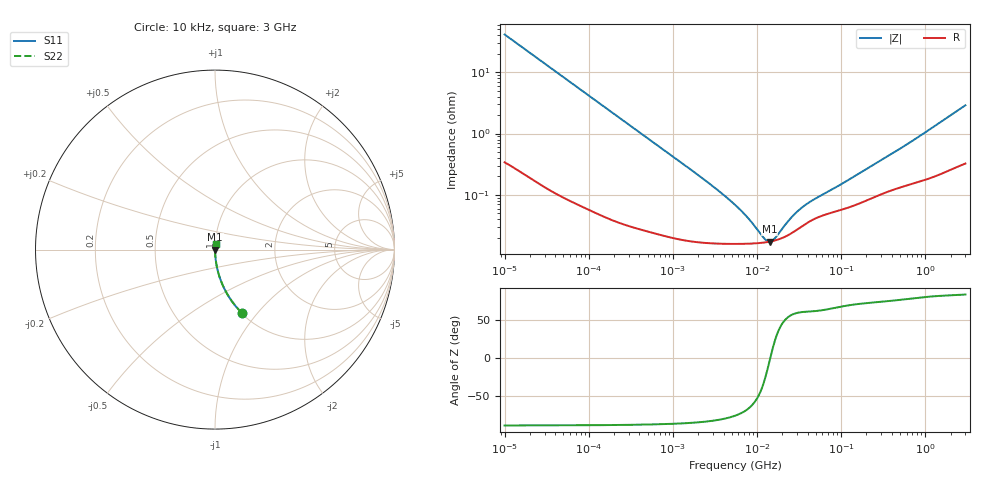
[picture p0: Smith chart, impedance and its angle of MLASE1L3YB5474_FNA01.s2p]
! MLASE1L3YB5474_FNA01  S-PARAMETER MODEL  ( Standard Model )
! Model Generated by TAIYO YUDEN Corporation (http://www.ty-top.com)
! Version 1.0
! TAIYO YUDEN Control No. 220601
! Copyright(c) 2010 TAIYO YUDEN CO.,LTD. All Rights Reserved.
! Product Description (link to TY-COMPAS)
! https://ds.yuden.co.jp/TYCOMPAS/or/detail?pn=MLASE1L3YB5474KFNA01&u=M
! Products Name : Multilayer Ceramic Capacitors
! Characteristics :
!  Capacitance : 0.47 [uF] , Rated Voltage : 16 [V] , TCC : X5R
!  Case Size : 1.0 x 0.5 / 0.039 x 0.02 [mm/inch] , Thickness : 0.3 / 0.012 [mm/inch]
!  (Conditions: Temperature = 25 [degC] , DC Bias Voltage = 0 [V])
! External Node Assignments :
!  1  o---| |---o  2
! GND o---------o GND
! Frequency Range : 10kHz  -  3GHz  [ 401 STEP ]
# MHZ S RI R 50
! Freq[MHz].  S11 Real  S11 Imag  S21 Real  S21 Imag  S12 Real  S12 Imag  S22 Real  S22 Imag
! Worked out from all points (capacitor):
!   401 points, 10 kHz to 3 GHz, reference 50 ohm
!   read as one part in series: C = 384 nF near 10.65 kHz
!   lowest |Z| = 17.3 mohm at 14.1 MHz (marker M1)
!   series resonance near 14.4 MHz, so ESL is about 320 pH
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0.01  0.148 -0.351  0.852 0.351  0.852 0.351  0.148 -0.351
0.016047  0.0645 -0.2412  0.9355 0.2412  0.9355 0.2412  0.0645 -0.2412
0.027426  0.0238 -0.1478  0.9762 0.1478  0.9762 0.1478  0.0238 -0.1478
0.045421  0.00929 -0.0908  0.9907 0.0908  0.9907 0.0908  0.00929 -0.0908
0.082683  0.00319 -0.0504  0.9968 0.0504  0.9968 0.0504  0.00319 -0.0504
0.199902  0.000819 -0.021  0.9992 0.021  0.9992 0.021  0.000819 -0.021
0.683653  0.000264 -0.0062  0.9997 0.0062  0.9997 0.0062  0.000264 -0.0062
2.652321  0.000166 -0.00156  0.9998 0.00156  0.9998 0.00156  0.000166 -0.00156
5.477226  0.000159 -0.000672  0.9998 0.000672  0.9998 0.000672  0.000159 -0.000672
7.996027  0.00016 -0.000373  0.9998 0.000373  0.9998 0.000373  0.00016 -0.000373
12.04705  0.000167 -0.000108  0.9998 0.000108  0.9998 0.000108  0.000167 -0.000108
13.24217  0.00017 -5.06e-05  0.9998 5.06e-05  0.9998 5.06e-05  0.00017 -5.06e-05
14.10408  0.000173 -1.26e-05  0.9998 1.26e-05  0.9998 1.26e-05  0.000173 -1.26e-05
15.02209  0.000176 2.54e-05  0.9998 -2.54e-05  0.9998 -2.54e-05  0.000176 2.54e-05
16.51234  0.000182 8.26e-05  0.9998 -8.26e-05  0.9998 -8.26e-05  0.000182 8.26e-05
23.35767  0.00022 0.000298  0.9998 -0.000298  0.9998 -0.000298  0.00022 0.000298
29.12589  0.000265 0.000439  0.9997 -0.000439  0.9997 -0.000439  0.000265 0.000439
36.31858  0.000325 0.000578  0.9997 -0.000578  0.9997 -0.000578  0.000325 0.000578
45.28751  0.000389 0.000712  0.9996 -0.000712  0.9996 -0.000712  0.000389 0.000712
102.7996  0.000578 0.00141  0.9994 -0.00141  0.9994 -0.00141  0.000578 0.00141
374.4521  0.00117 0.00429  0.9988 -0.00429  0.9988 -0.00429  0.00117 0.00429
3000  0.00405 0.0285  0.9959 -0.0285  0.9959 -0.0285  0.00405 0.0285
